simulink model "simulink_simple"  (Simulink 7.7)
settings: Solver=ode15s  StartTime=0.0  StopTime=24  RelTol=1e-3
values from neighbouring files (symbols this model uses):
  A = [((-UAfr)/mCpf) (UAfr/mCpf) 0; (UAfr/mCpr) ((-UAro-UAfr)/mCpr) 0; 0 0 0]    [simplemodel.m]
  B = [1/mCpf 0 0 ; 0 1/mCpr (UAro/mCpr); 0 1 0]    [simplemodel.m]
  C = [1 0 0; 0 1 0; 0 0 1]    [simplemodel.m]
  D = [0 0 0 ; 0 0 0; 0 0 0]    [simplemodel.m]
  init = [Tf Tr E]    [simplemodel.m]
  qhf = 0    [simplemodel.m]
  qhr = 4000*60*60    (= 14400000)    [simplemodel.m]
  To = 273+0    (= 273)    [simplemodel.m]

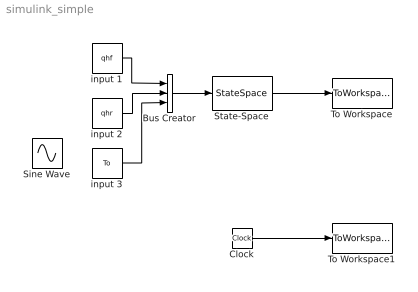
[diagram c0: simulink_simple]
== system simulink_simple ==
  Bus Creator : BusCreator  Inputs=3
  Clock : Clock
  Sine Wave : Sin  SampleTime=0
  State-Space : StateSpace  A=A  B=B  C=C  D=D  X0=init
  To Workspace : ToWorkspace  VariableName=simout  SampleTime=-1  SaveFormat=Array
  To Workspace1 : ToWorkspace  VariableName=time  SampleTime=-1  SaveFormat=Array
  input 1 : Constant  Value=qhf
  input 2 : Constant  Value=qhr
  input 3 : Constant  Value=To
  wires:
  input 1/1 -> Bus Creator/1
  input 2/1 -> Bus Creator/2
  Bus Creator/1 -> State-Space/1
  State-Space/1 -> To Workspace/1
  input 3/1 -> Bus Creator/3
  Clock/1 -> To Workspace1/1
